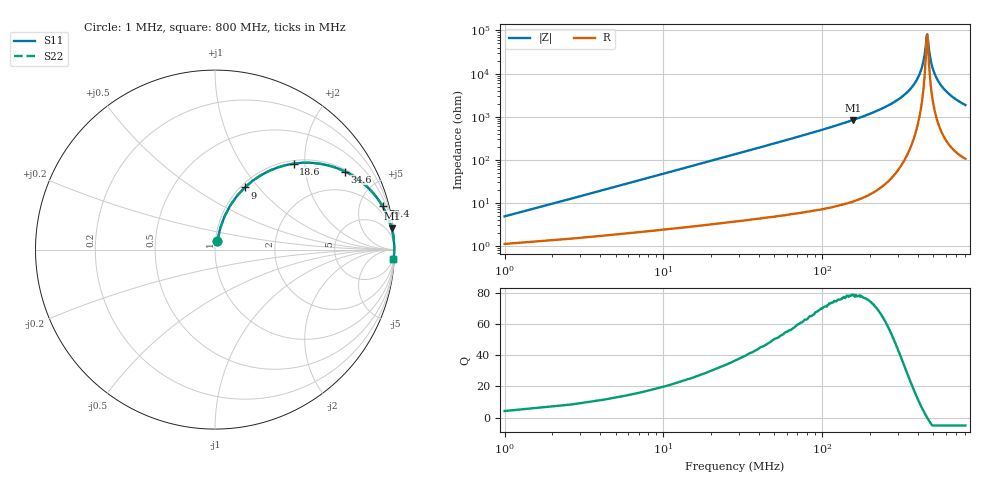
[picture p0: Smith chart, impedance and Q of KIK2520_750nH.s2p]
!version-2
!date-01.2022
!Series
# MHz S RI R 50
!Freq ReS11 ImS11 ReS21 ImS21 ReS12 ImS12 ReS22 ImS22
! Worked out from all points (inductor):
!   501 points, 1 MHz to 800 MHz, reference 50 ohm
!   read as one part in series: L = 750 nH near 4.2 MHz
!   highest Q = 78.4 at 156 MHz (marker M1), where L = 849 nH
!   self-resonance near 459 MHz
!   S11 on the Smith chart (normalised r, x): 1 MHz: 1.02, +0.09; 9 MHz: 1.05, +0.85; 18.6 MHz: 1.06, +1.76; 34.6 MHz: 1.08, +3.28; 79.4 MHz: 1.12, +7.71; 800 MHz: 3, -37
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1  0.0131 0.046  0.9869 -0.046  0.9869 -0.046  0.0131 0.046
5.8  0.0848 0.2454  0.9152 -0.2454  0.9152 -0.2454  0.0848 0.2454
9  0.1658 0.346  0.8342 -0.346  0.8342 -0.346  0.1658 0.346
18.6  0.4377 0.479  0.5623 -0.479  0.5623 -0.479  0.4377 0.479
34.6  0.7242 0.4349  0.2758 -0.4349  0.2758 -0.4349  0.7242 0.4349
52.2  0.8565 0.3409  0.1435 -0.3409  0.1435 -0.3409  0.8565 0.3409
79.4  0.9337 0.241  0.0663 -0.241  0.0663 -0.241  0.9337 0.241
135  0.9782 0.1397  0.0218 -0.1397  0.0218 -0.1397  0.9782 0.1397
156  0.9843 0.1181  0.0157 -0.1181  0.0157 -0.1181  0.9843 0.1181
268  0.9964 0.0519  0.00365 -0.0519  0.00365 -0.0519  0.9964 0.0519
347  0.9983 0.0263  0.00165 -0.0263  0.00165 -0.0263  0.9983 0.0263
401  0.9988 0.0126  0.00122 -0.0126  0.00122 -0.0126  0.9988 0.0126
435  0.9988 0.00514  0.00118 -0.00514  0.00118 -0.00514  0.9988 0.00514
446  0.9988 0.0028  0.00119 -0.0028  0.00119 -0.0028  0.9988 0.0028
455  0.9988 0.000832  0.00121 -0.000832  0.00121 -0.000832  0.9988 0.000832
460  0.9988 -0.000134  0.00123 0.000134  0.00123 0.000134  0.9988 -0.000134
476  0.9987 -0.00328  0.00129 0.00328  0.00129 0.00328  0.9987 -0.00328
487  0.9986 -0.00542  0.00135 0.00542  0.00135 0.00542  0.9986 -0.00542
534  0.9983 -0.0138  0.0017 0.0138  0.0017 0.0138  0.9983 -0.0138
591  0.9977 -0.0234  0.00232 0.0234  0.00232 0.0234  0.9977 -0.0234
667  0.9966 -0.0349  0.0034 0.0349  0.0034 0.0349  0.9966 -0.0349
800  0.9941 -0.0533  0.00589 0.0533  0.00589 0.0533  0.9941 -0.0533
